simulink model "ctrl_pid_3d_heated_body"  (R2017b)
settings: Solver=ode45  StartTime=0.0  StopTime=70  RelTol=1e-3
libraries: dps x8

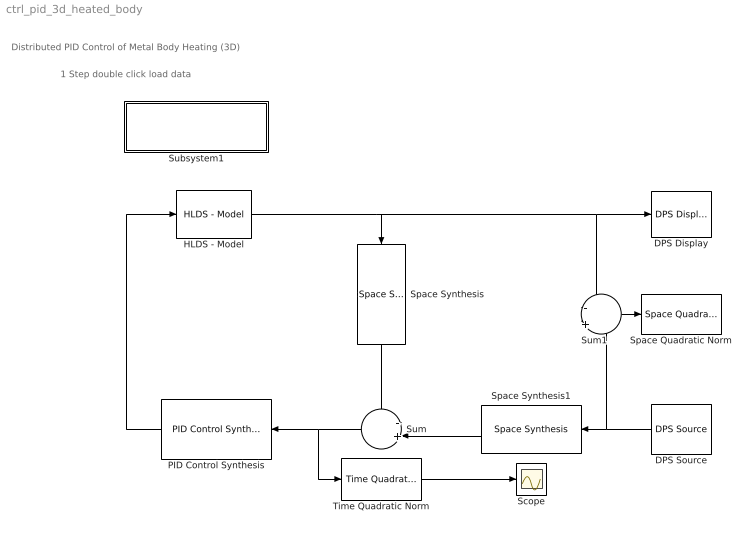
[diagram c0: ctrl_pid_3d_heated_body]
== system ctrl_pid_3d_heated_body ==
  note: Distributed PID Control of Metal Body Heating (3D)
  note: 1 Step double click load data
  DPS Display : dps/DPS Display  graphType=surf  pointCoord=M  elementsVar=e  showColor=on  minC=0  maxC=350  showDeform=off  deform=z  deformScale=0.001  showScope=off  responseVar=H  aviparam=0
  DPS Source : dps/DPS Source  equation='300*ones(size(x))'  responseVar=0  showInput=on  pointsCoord=M  elementsVar=e  samplePeriod=1
  HLDS - Model : dps/Controlled Systems/HLDS - Model  StepResponse=H  samplePeriod=1  u_step=1
  PID Control Synthesis : dps/Temporal Synthesis/PID Control Synthesis  method=Manual  r0=[0.00082,0.00082,0.00097,0.00124]  ri=[0.00034,0.00034,0.00037,0.00057]  rd=[0, 0, 0, 0]  b=[]  a=[]  tau=[]  StepResponse=H  weights=[]  samplePeriod=1
  Scope : Scope
  Space Quadratic Norm : dps/Quadratic norms/Space Quadratic Norm  StepResponse=H  showNorm=on
  Space Synthesis : dps/Space Synthesis/Space Synthesis  PCH=H  weights=[]
  Space Synthesis1 : dps/Space Synthesis/Space Synthesis  PCH=H  weights=[]
  Subsystem1 : Subsystem
  Sum : Sum  Inputs=-+|
  Sum1 : Sum  Inputs=-|+
  Time Quadratic Norm : dps/Quadratic norms/Time Quadratic Norm
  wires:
  Sum/1 -> Time Quadratic Norm/1, PID Control Synthesis/1
  DPS Source/1 -> Sum1/2, Space Synthesis1/1
  PID Control Synthesis/1 -> HLDS - Model/1
  HLDS - Model/1 -> DPS Display/1, Sum1/1, Space Synthesis/1
  Space Synthesis1/1 -> Sum/2
  Space Synthesis/1 -> Sum/1
  Time Quadratic Norm/1 -> Scope/1
  Sum1/1 -> Space Quadratic Norm/1

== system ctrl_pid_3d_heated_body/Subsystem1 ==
